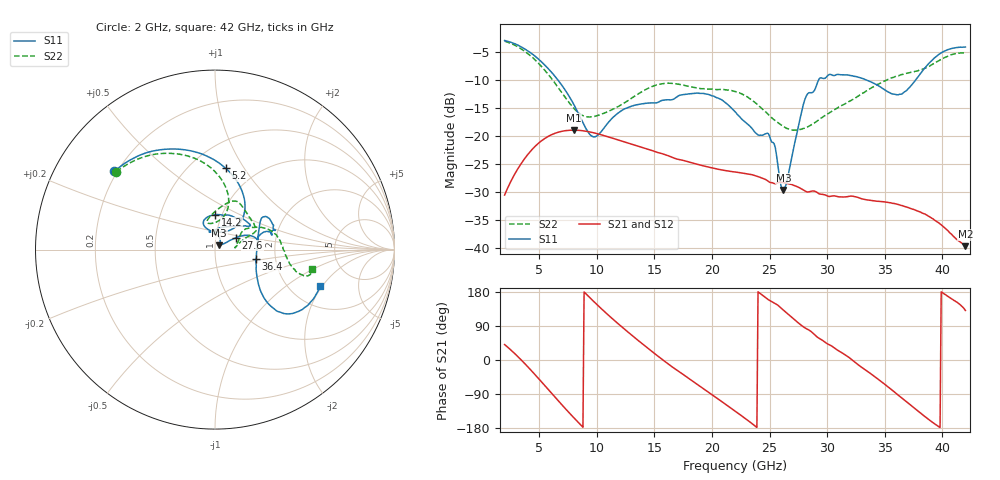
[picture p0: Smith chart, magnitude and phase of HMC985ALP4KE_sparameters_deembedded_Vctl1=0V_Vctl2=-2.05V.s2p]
!s2p File: Measurements: S11, S21, S12, S22
# GHz S dB R 50.0
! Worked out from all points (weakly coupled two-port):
!   401 points, 2 GHz to 42 GHz, reference 50 ohm
!   highest |S21| = -19.00 dB at 8 GHz (marker M1); lowest = -39.7 dB at 42 GHz (marker M2)
!   lowest |S11| = -29.7 dB at 26.2 GHz (marker M3), VSWR 1.07, Z = 52.3 + j2.4 ohm
!   |S11| at or under -10 dB: 6.613 GHz to 29.27 GHz (22.65 GHz wide, 126 % of centre); 33.37 GHz to 37.7 GHz (4.33 GHz wide, 12.2 % of centre)
!   |S22| runs from -19.0 to -3.1 dB; largest |S21 - S12| = 0.00015
!   S11 on the Smith chart (normalised r, x): 2 GHz: 0.19, +0.33; 5.2 GHz: 0.72, +0.83; 14.2 GHz: 0.93, +0.38; 27.6 GHz: 1.25, +0.17; 36.4 GHz: 1.58, -0.18; 42 GHz: 2.90, -1.91
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2  -2.97 142.1  -30.60 40.8  -30.60 40.8  -3.10 141.7
3.6  -4.31 112.9  -24.49 -4.8  -24.49 -4.8  -4.71 113.1
5.2  -6.79 82.6  -20.91 -57.6  -20.91 -57.6  -7.62 87.6
8  -14.38 47.2  -19.00 -152.1  -19.00 -152.1  -15.08 77.9
8.7  -17.27 52.2  -19.09 -174.2  -19.09 -174.2  -16.30 87.7
9.9  -20.15 89.5  -19.56 149.6  -19.56 149.6  -16.49 103.2
12.1  -15.58 112.9  -20.90 89.3  -20.91 89.3  -14.49 98.0
14.2  -14.22 89.7  -22.25 36.7  -22.25 36.7  -11.79 77.9
15.4  -13.94 73.2  -23.05 8.3  -23.06 8.3  -10.81 69.9
19.3  -12.45 34.3  -25.40 -76.6  -25.40 -76.6  -11.59 41.2
22  -15.70 52.3  -26.48 -134.5  -26.48 -134.5  -12.09 24.3
25  -20.06 98.5  -28.30 157.3  -28.31 157.3  -16.43 17.0
26.2  -29.70 44.4  -28.38 131.6  -28.38 131.6  -18.35 8.9
27.6  -17.39 29.7  -29.30 95.3  -29.30 95.4  -18.88 6.5
28.1  -13.32 20.9  -29.89 84.3  -29.90 84.2  -18.61 9.3
28.7  -12.28 13.0  -29.88 72.8  -29.88 72.7  -17.95 14.4
31  -9.06 23.3  -30.92 24.2  -30.91 24.2  -14.89 33.5
33.3  -9.94 34.2  -31.42 -25.6  -31.41 -25.7  -12.16 30.0
35.4  -12.27 12.1  -31.97 -73.8  -31.95 -73.9  -9.85 20.0
36.4  -12.58 -13.0  -32.45 -98.3  -32.44 -98.3  -9.09 13.7
39.5  -5.81 -43.4  -35.34 -171.8  -35.32 -171.8  -6.79 -14.0
42  -4.14 -19.0  -39.74 130.6  -39.71 130.9  -5.22 -11.1
